{attribute 'qualified_only'}
VAR_GLOBAL
 
	
	
	
	
	
	ActiveScenes_byte0_port1 AT %Q* : USINT;
	ActiveScenes_byte1_port1 AT %Q* : USINT;
	
    Number_byte0_port1 AT %Q* : USINT;
    Number_byte1_port1 AT %Q* : USINT;
    Number_byte2_port1 AT %Q* : USINT;
    Number_byte3_port1 AT %Q* : USINT;
	
	String_byte0_port1 AT %Q* : USINT;
	String_byte1_port1 AT %Q* : USINT;
	String_byte2_port1 AT %Q* : USINT;
	String_byte3_port1 AT %Q* : USINT;
	String_byte4_port1 AT %Q* : USINT;
	String_byte5_port1 AT %Q* : USINT;
	
	caneoSeries52_PDin_port1 : series5x_PDin;
	caneoSeries52_PDout_port1: series5x_PDout;
	
	//mapping for variables to io link process data
	//PD out
	//processdata[15] = mode
	//processdata[13] = ActiveScenes_byte1_port1
	//processdata[12] = ActiveScenes_byte0_port1
	//processdata[11] = Number_byte3_port1
	//processdata[10] = Number_byte2_port1
	//processdata[9] = Number_byte1_port1
	//processdata[8] = Number_byte0_port1
	//processdata[7]= textselect
	//processdata[6] = color
	//processdata[5] = String_byte5_port1
	//processdata[4] = String_byte4_port1
	//processdata[3] = String_byte3_port1
	//processdata[2] = String_byte2_port1
	//processdata[1] = String_byte1_port1
	//processdata[0] = String_byte0_port1
	
	
	
END_VAR
